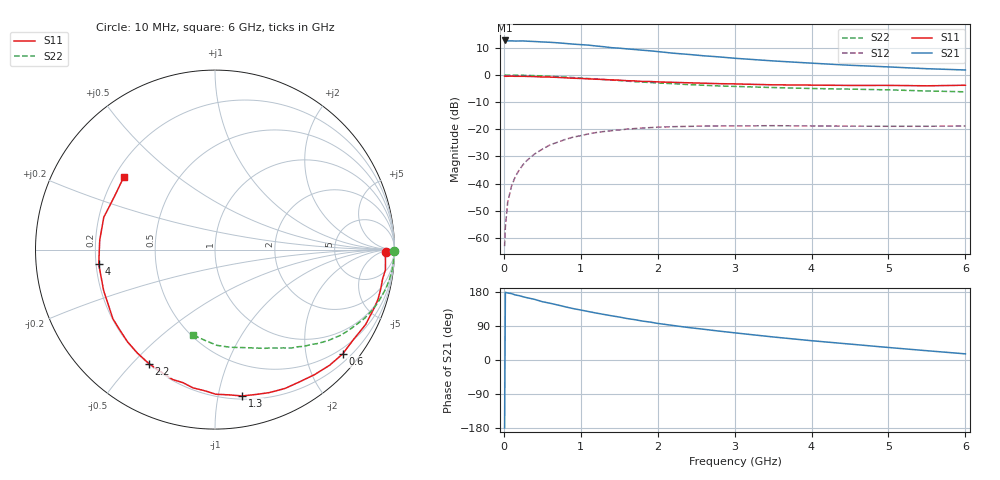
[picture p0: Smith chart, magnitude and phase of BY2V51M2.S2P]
! SIEMENS Small Signal Semiconductors
! BFY420
! Si NPN RF SIEGET Grounded Emitter Transistor in MICRO-X
! VCE = 2.5 V  IC = 1.2 mA
! Common Emitter S-Parameters:  October  1996
# GHz  S  MA  R  50
!  f  S11  S21  S12  S22
! GHz  MAG  ANG  MAG  ANG  MAG  ANG  MAG  ANG
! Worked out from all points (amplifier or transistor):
!   36 points, 10 MHz to 6 GHz, reference 50 ohm
!   highest |S21| = 12.8 dB at 10 MHz (marker M1)
!   |S21| within 3 dB of that: start of sweep to 1.559 GHz
!   unconditionally stable (mu >= 1): 4.404 GHz to end of sweep
!   at 250 MHz: K = 0.04, MSG = 22.8 dB, |S12| = -33.0 dB
!   at 1.4 GHz: K = 0.22, MSG = 15.3 dB, |S12| = -20.5 dB
!   at 6 GHz: K = 1.31, MAG = 7.0 dB, |S12| = -18.8 dB
!   S11 on the Smith chart (normalised r, x): 10 MHz: 40, -10; 600 MHz: 0.37, -2.76; 1.3 GHz: 0.23, -1.18; 2.2 GHz: 0.20, -0.56; 4 GHz: 0.21, -0.06; 6 GHz: 0.24, +0.33
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0.01  0.9542 -0.7  4.347 -179.4  0.0007 111.2  0.9993 -0.3
0.02  0.949 -1.7  4.319 178.6  0.0016 91.8  0.9999 -0.7
0.05  0.9512 -3.3  4.264 176.9  0.0045 85.0  0.9973 -1.6
0.1  0.9563 -6.8  4.276 175.2  0.009 87.4  0.9966 -3.3
0.15  0.9479 -9.9  4.24 171.6  0.0135 83.7  0.9949 -4.9
0.2  0.9491 -13.3  4.251 169.8  0.0178 83.1  0.9939 -6.4
0.25  0.9496 -16.8  4.261 166.9  0.0223 79.6  0.9895 -8.0
0.4  0.9375 -26.4  4.156 160.0  0.0351 74.0  0.9766 -12.8
0.5  0.9203 -32.8  4.08 153.9  0.043 70.4  0.964 -15.8
0.6  0.9185 -39.3  4.02 149.8  0.0515 66.7  0.9504 -18.8
0.8  0.8906 -51.4  3.828 140.3  0.0651 59.0  0.9177 -24.6
1.1  0.8522 -69.2  3.563 127.9  0.0822 49.6  0.8628 -32.1
1.3  0.8293 -79.5  3.328 120.3  0.091 43.9  0.8262 -36.6
1.8  0.7625 -103.6  2.876 102.8  0.1053 31.9  0.7431 -45.9
2.2  0.7345 -120.0  2.532 91.1  0.1118 24.2  0.6935 -52.3
2.4  0.7205 -126.9  2.405 85.7  0.1133 21.6  0.6669 -55.2
2.8  0.6939 -140.0  2.162 76.2  0.1156 16.3  0.6295 -60.4
3.5  0.6609 -159.9  1.824 60.8  0.1166 9.7  0.5885 -68.6
4  0.6529 -172.8  1.658 50.9  0.1155 6.7  0.5655 -74.8
4.5  0.6444 175.3  1.517 42.0  0.1141 4.3  0.5507 -81.2
5.5  0.6337 152.1  1.31 24.5  0.1137 2.9  0.5094 -96.1
6  0.6492 141.6  1.241 16.2  0.1149 3.7  0.4909 -104.7
